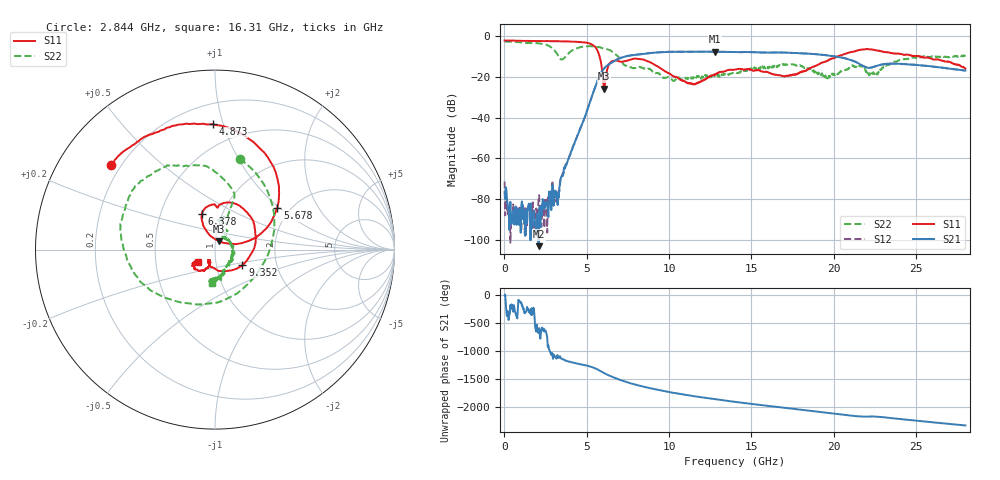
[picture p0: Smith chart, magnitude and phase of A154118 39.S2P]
!  2-Port S-parameters saved by WinCal
! VAR MeasName=S-Parameters (CALIBRATED_DATA) read from VNA (N5230A)
! VAR MeasDate=2015-9-10 14:37:25
! VAR NAME=A154118 39
! VAR FILENAME=A154118 39.S2P
! VAR DATE=2015-9-10 14:37:25
! VAR PHYS_PORTS=1,2
# Hz S DB R 50
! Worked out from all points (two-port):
!   801 points, 10 MHz to 28 GHz, reference 50 ohm
!   highest |S21| = -7.65 dB at 12.78 GHz (marker M1); lowest = -103.1 dB at 2.074 GHz (marker M2)
!   |S21| within 3 dB of the highest: 7.08 GHz to 20.55 GHz (13.47 GHz wide, 97.5 % of centre)
!   lowest |S11| = -25.8 dB at 6.063 GHz (marker M3), VSWR 1.11, Z = 51.8 + j4.9 ohm
!   |S11| at or under -10 dB: 5.781 GHz to 20.25 GHz (14.47 GHz wide, 111 % of centre); 25.19469 GHz to 25.20741 GHz (12.72 MHz wide, 0.0505 % of centre); 25.26 GHz to end of sweep
!   |S22| runs from -22.0 to -2.7 dB; largest |S21 - S12| = 0.0082
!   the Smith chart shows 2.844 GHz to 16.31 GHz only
!   S11 on the Smith chart (normalised r, x): 2.844 GHz: 0.16, +0.35; 4.873 GHz: 0.34, +0.92; 5.678 GHz: 1.72, +0.97; 6.378 GHz: 0.80, +0.33; 9.352 GHz: 1.34, -0.24; 16.31 GHz: 0.82, -0.11
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1e7  -2.15 179.7  -76.47 -10.9  -71.32 -162.8  -2.67 179.8
2.899e8  -2.19 175.7  -95.07 2.2  -88.90 115.4  -2.71 172.9
2.074262e9  -2.43 152.5  -103.11 34.7  -79.35 101.0  -3.54 125.0
2.843988e9  -2.52 141.0  -85.39 9.4  -80.64 45.1  -5.58 74.7
3.193862e9  -2.51 134.9  -77.08 -1.8  -79.41 -33.5  -8.71 25.6
3.683688e9  -2.63 125.1  -65.00 -91.6  -64.61 -88.6  -10.42 -95.5
4.698325e9  -3.02 98.1  -43.50 -164.2  -43.57 -163.6  -5.32 166.0
4.873262e9  -3.12 91.0  -40.06 -173.4  -40.05 -173.4  -5.24 157.7
5.677975e9  -7.58 33.8  -21.38 106.0  -21.31 106.1  -5.39 121.1
6.062838e9  -25.82 67.1  -15.78 43.5  -15.71 43.5  -6.23 107.6
6.377725e9  -13.54 110.1  -13.71 -1.5  -13.65 -1.6  -6.83 93.9
7.392362e9  -12.17 85.2  -9.89 -112.7  -9.89 -113.0  -14.49 69.8
8.302038e9  -11.36 45.0  -8.89 172.7  -8.86 172.5  -15.26 79.1
9.351662e9  -15.11 -29.5  -8.05 104.2  -7.96 104.1  -18.28 59.4
1.103106e10  -22.54 -120.0  -7.68 14.8  -7.64 14.4  -20.93 37.7
1.278044e10  -18.78 -114.0  -7.65 -60.8  -7.63 -61.4  -18.97 -35.5
1.4005e10  -16.45 -132.4  -7.85 -108.0  -7.82 -108.6  -18.14 -65.1
1.631418e10  -18.63 -145.4  -8.07 170.9  -8.07 170.4  -14.62 -95.5
1.869332e10  -15.21 -104.3  -8.76 88.6  -8.77 88.2  -16.36 -130.4
2.121242e10  -7.62 -126.3  -12.24 1.7  -12.19 0.4  -14.76 -102.8
2.334666e10  -8.07 -168.3  -13.53 -32.3  -13.53 -33.8  -14.01 -80.9
2.8e10  -15.99 161.1  -16.91 -168.3  -17.00 -169.3  -9.34 -118.3
